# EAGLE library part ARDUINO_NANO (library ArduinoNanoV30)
Arduino Nano V3.0 Overview: The Arduino Nano is a small, complete, and breadboard-friendly board based on the ATmega328 (Arduino Nano 3.x) or ATmega168 (Arduino Nano 2.x). It has more or less the same functionality of the Arduino Duemilanove, but in a different package. It lacks only a DC power jack, and works with a Mini-B USB cable instead of a standard one. The Nano was designed and is being produced by Gravitech. Specifications: Microcontroller Atmel ATmega168 or ATmega328 Operating Voltage (logic level) 5 V Input Voltage (recommended) 7-12 V Input Voltage (limits) 6-20 V Digital I/O Pins 14 (of which 6 provide PWM output) Analog Input Pins 8 DC Current per I/O Pin 40 mA Flash Memory 16 KB (ATmega168) or 32 KB (ATmega328) of which 2 KB used by bootloader SRAM 1 KB (ATmega168) or 2 KB (ATmega328) EEPROM 512 bytes (ATmega168) or 1 KB (ATmega328) Clock Speed 16 MHz Dimensions 0.73" x 1.70" Length 45 mm Width 18 mm Weigth 5 g Power: The Arduino Nano can be powered via the Mini-B USB connection, 6-20V unregulated external power supply (pin 30), or 5V regulated external power supply (pin 27). The power source is automatically selected to the highest voltage source. Memory: The ATmega168 has 16 KB of flash memory for storing code (of which 2 KB is used for the bootloader); the ATmega328 has 32 KB, (also with 2 KB used for the bootloader). The ATmega168 has 1 KB of SRAM and 512 bytes of EEPROM (which can be read and written with the EEPROM library); the ATmega328 has 2 KB of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
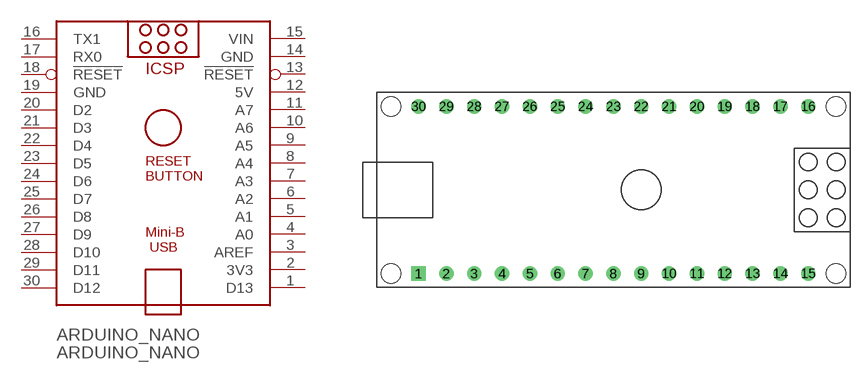
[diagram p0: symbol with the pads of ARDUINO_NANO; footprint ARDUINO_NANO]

Designator prefix ARDUINO_NANO

## ARDUINO_NANO  [ARDUINO_NANO]
1  D13
2  3V3  out
3  AREF  in
4  A0
5  A1
6  A2
7  A3
8  A4
9  A5
10  A6
11  A7
12  5V  pwr
13  !RESET  in
14  GND  pwr
15  VIN  pwr
16  TX1
17  RX0
18  !RESET  in
19  GND  pwr
20  D2
21  D3
22  D4
23  D5
24  D6
25  D7
26  D8
27  D9
28  D10
29  D11
30  D12

## Footprint ARDUINO_NANO (pad centres in mm)
Arduino Nano V3.0 The Nano was designed and is being produced by Gravitech. Gravitech Arduino Nano V3.0
drill 0.8 square: 1 -20.32,-7.62
drill 0.8: 2 -17.78,-7.62; 3 -15.24,-7.62; 4 -12.7,-7.62; 5 -10.16,-7.62; 6 -7.62,-7.62; 7 -5.08,-7.62; 8 -2.54,-7.62; 9 0,-7.62; 10 2.54,-7.62; 11 5.08,-7.62; 12 7.62,-7.62; 13 10.16,-7.62; 14 12.7,-7.62; 15 15.24,-7.62; 16 15.24,7.62; 17 12.7,7.62; 18 10.16,7.62; 19 7.62,7.62; 20 5.08,7.62; 21 2.54,7.62; 22 0,7.62; 23 -2.54,7.62; 24 -5.08,7.62; 25 -7.62,7.62; 26 -10.16,7.62; 27 -12.7,7.62; 28 -15.24,7.62; 29 -17.78,7.62; 30 -20.32,7.62
hole 1.778 at -22.86,-7.62
hole 1.778 at -22.86,7.62
hole 1.778 at 17.78,7.62
hole 1.778 at 17.78,-7.62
